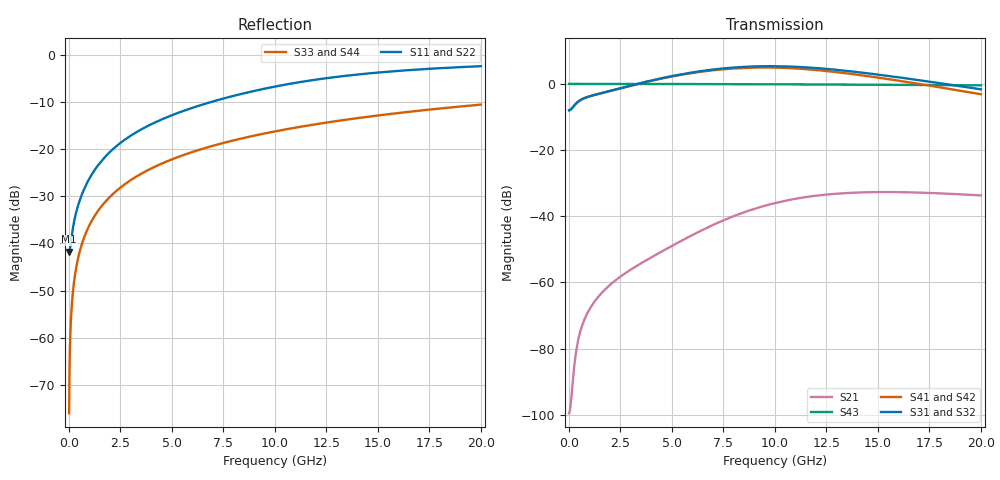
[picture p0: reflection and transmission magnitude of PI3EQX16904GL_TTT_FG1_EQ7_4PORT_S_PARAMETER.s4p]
! NPort=4 DATA=2000 NOISE=0 GROUPDELAY=0 COMPLEX_DATAFORMAT=POLAR
! NumOfBlock=1 NumOfParam=0
! .MODEL Smodel S TSTONEFILE=PI3EQX16904GL_TTT_FG1_EQ7_4PORT_S_PARAMETER.s4p TYPE=S
!  -- The above .MODEL line can be used for the S element in the netlist.
! The s parameter is extracted from the linear redriver, it is not bi-directional; only s(4,1)s(4,2) and s(3,1)s(3,2)
! should be the insertion loss
!Port definition:
!Port1 = input+
!Port2 = input-
!Port3 = output+
!Port4 = output-
# Hz S MA R  50
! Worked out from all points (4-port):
!   2000 points, 10 MHz to 20 GHz, reference 50 ohm
!   strongest paths, dB at 10 MHz, 5.01 GHz, 10.01 GHz, 15.01 GHz, 20 GHz:
!     S31: -8.0, 2.4, 5.4, 2.8, -1.6
!     S32: -8.0, 2.3, 5.3, 2.7, -1.8
!     S41: -8.0, 2.3, 4.9, 1.9, -3.1
!     S42: -8.0, 2.2, 4.9, 1.8, -3.3
!     S43: 0.0, 0.0, -0.1, -0.3, -0.4
!     S21: -99.6, -48.9, -36.0, -32.7, -33.7
!   lowest |S11| = -41.7 dB at 10 MHz (marker M1), VSWR 1.02, Z = 49.2 - j0.0603 ohm
!   |S11| at or under -10 dB: start of sweep to 6.858 GHz
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1e7  0.008182 -175.7  1.05e-05 7.8  0 0.0  0 0.0
     1.05e-05 7.8  0.008182 -175.7  0 0.0  0 0.0
     0.3996 0.7  0.3996 -179.3  0.0001571 -90.0  1 -0.0
     0.3996 -179.3  0.3996 0.7  1 -0.0  0.0001571 -90.0
3.8e8  0.02256 -119.7  0.0001026 118.5  0 0.0  0 0.0
       0.0001026 118.5  0.02256 -119.7  0 0.0  0 0.0
       0.5174 15.2  0.5175 -164.9  0.005969 -90.4  1 -0.3
       0.5173 -165.5  0.5174 14.5  1 -0.3  0.005969 -90.4
1.57e9  0.07465 -102.9  0.0006817 110.7  0 0.0  0 0.0
        0.0006813 110.7  0.07465 -102.9  0 0.0  0 0.0
        0.7248 9.3  0.726 -170.8  0.02465 -91.5  0.9997 -1.4
        0.7239 -173.5  0.7251 6.4  0.9997 -1.4  0.02465 -91.5
5.78e9  0.266 -104.3  0.00484 109.4  0 0.0  0 0.0
        0.004803 109.8  0.2659 -104.3  0 0.0  0 0.0
        1.454 -34.4  1.445 145.0  0.09039 -95.4  0.9956 -5.2
        1.43 135.3  1.421 -45.2  0.9956 -5.2  0.09039 -95.4
9.41e9  0.4368 -111.2  0.01422 75.1  0 0.0  0 0.0
        0.01413 76.0  0.4367 -111.2  0 0.0  0 0.0
        1.85 -95.9  1.835 83.6  0.1461 -98.7  0.9884 -8.4
        1.772 67.7  1.757 -112.8  0.9884 -8.4  0.1461 -98.7
1.339e10  0.6026 -121.8  0.0224 23.2  0 0.0  0 0.0
          0.02231 24.6  0.6027 -121.8  0 0.0  0 0.0
          1.585 -163.6  1.569 15.8  0.2055 -102.3  0.9769 -11.9
          1.457 -6.4  1.442 173.1  0.9769 -11.9  0.2055 -102.3
2e10  0.7645 -136.5  0.02064 -38.7  0 0.0  0 0.0
      0.02066 -36.5  0.765 -136.5  0 0.0  0 0.0
      0.8288 107.4  0.8163 -73.3  0.2986 -108.1  0.9506 -17.4
      0.6978 -104.6  0.6873 74.8  0.9506 -17.4  0.2986 -108.1
